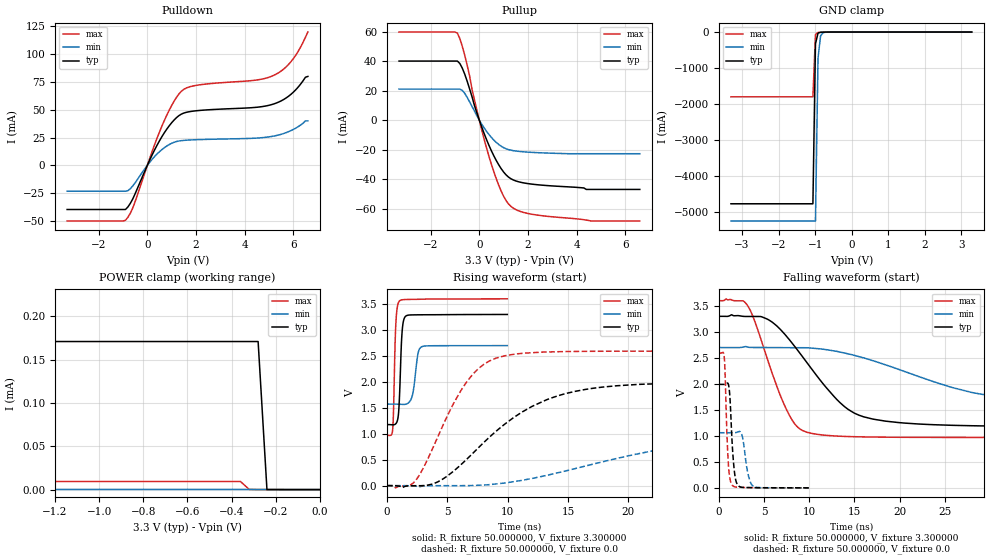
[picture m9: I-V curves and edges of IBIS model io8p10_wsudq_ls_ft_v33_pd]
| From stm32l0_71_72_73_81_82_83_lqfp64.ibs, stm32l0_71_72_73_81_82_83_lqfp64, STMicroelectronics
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|   Model io8p10_wsudq_ls_ft_v33_pd
[Model]  io8p10_wsudq_ls_ft_v33_pd
Model_type I/O
Polarity   Non-Inverting
Enable   Active-Low
Vinl =   0.990000V
Vinh =   2.310000V
Vmeas =  1.650000V
Cref =   50.000000pF
Rref =   100.000000M
Vref =   0.0V
C_comp   2.653200pF   2.620200pF   2.695100pF
[Temperature Range]   25.000000   0.125000k   -40.000000
[Pullup Reference]   3.300000V   2.700000V   3.600000V
[Pulldown Reference]   0.0V   0.0V   0.0V
[POWER Clamp Reference]   3.300000V   2.700000V   3.600000V
[GND Clamp Reference]   0.0V   0.0V   0.0V
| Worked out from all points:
|   slope of the pulldown table from 0 to 0.495 V, typ, clamps not added: 22.6 ohm
|   slope of the pullup table from 0 to 0.495 V, typ, clamps not added: 23.9 ohm
|   GND clamp passes 1 mA (typ) near -0.64 V on its own axis
|   POWER clamp passes 1 mA (typ) near -2.99 V on its own axis
|   rising waveform, R_fixture 50.000000, V_fixture 3.300000: 20-80 % time 213ps typ, 360ps min, 178ps max; typ from 1.18 V to 3.3 V
|   rising waveform, R_fixture 50.000000, V_fixture 0.0: 20-80 % time 6.53ns typ, 13.6ns min, 3.46ns max; typ from 0 V to 1.99 V
|   falling waveform, R_fixture 50.000000, V_fixture 3.300000: 20-80 % time 5.97ns typ, 12.7ns min, 3.28ns max; typ from 3.3 V to 1.18 V
|   falling waveform, R_fixture 50.000000, V_fixture 0.0: 20-80 % time 397ps typ, 565ps min, 319ps max; typ from 1.99 V to 0 V
[Pulldown]
|Voltage   I(typ)   I(min)   I(max)
-3.3V     -39.83mA   -23.37mA   -50.2mA
-900mV    -39.83mA   -23.37mA   -49.53mA
-600mV    -30.28mA   -18.59mA   -38.45mA
100mV     4.867mA    2.821mA    6.48mA
600mV     25.85mA    14.17mA    35.39mA
1V        38.33mA    19.81mA    53.88mA
1.4V      46.1mA     22.18mA    66.72mA
2V        49.07mA    23.02mA    71.93mA
4.4V      52.05mA    24.38mA    76.53mA
5.2V      55.25mA    26.3mA     81.02mA
5.9V      63.83mA    31.17mA    93.18mA
6.6V      80mA       40mA       120mA
[Pullup]
|Voltage   I(typ)   I(min)   I(max)
-3.3V     40.01mA    21.01mA    59.69mA
-900mV    40.01mA    21.01mA    58.93mA
-800mV    38.37mA    21.01mA    55.25mA
-600mV    31.19mA    18.18mA    44.04mA
0V        0A         0A         0A
500mV     -20.88mA   -11.78mA   -30.07mA
900mV     -32.92mA   -17.72mA   -48.15mA
1.3V      -39.75mA   -20.4mA    -58.47mA
1.8V      -42.5mA    -21.48mA   -62.49mA
2.7V      -44.27mA   -22.29mA   -65.04mA
4.6V      -47mA      -22.8mA    -68.41mA
6.6V      -47mA      -22.8mA    -68.41mA
[GND_clamp]
|Voltage   I(typ)   I(min)   I(max)
-3.3V     -4.766A    -5.244A    -1.797A
-1.06V    -4.766A    -5.244A    -1.797A
-990mV    -326.8mA   -5.244A    -68.06mA
-920mV    -29.1mA    -722.2mA   -11.17mA
-850mV    -6.81mA    -104.4mA   -6.691mA
-780mV    -3.567mA   -17.46mA   -4.273mA
-500mV    -68.7uA    -184.5uA   -41.56uA
3.28V     73.95uA    88.62uA    51.48uA
[POWER_clamp]
|Voltage   I(typ)   I(min)   I(max)
-3.28V    3.05A      15.65uA    3.723A
-3.2V     3.05A      1.687uA    3.723A
-2.96V    269.4uA    209.1nA    3.723A
-2.92V    170.9uA    209.1nA    508.5mA
-2.8V     170.9uA    209.1nA    1.296mA
-2.76V    170.9uA    209.1nA    177.1uA
-2.72V    170.9uA    209.1nA    24.25uA
-2.68V    170.9uA    209.1nA    9.362uA
-360mV    170.9uA    209.1nA    9.362uA
-280mV    170.9uA    209.1nA    0A
-240mV    0A         209.1nA    0A
0V        0A         0A         0A
[Ramp]
| variable   typ   min   max
dV/dt_r  1.19406/6.52281n   0.62958/13.57033n   1.55520/3.45923n
dV/dt_f  1.27356/5.95863n   0.65610/12.61269n   1.57835/3.27280n
R_load = 50.000000
[Rising Waveform]
R_fixture= 50.000000
V_fixture= 3.300000
V_fixture_min= 2.700000
V_fixture_max= 3.600000
|time   V(typ)   V(min)   V(max)
0s        1.176V     1.571V     968.9mV
480.5ps   1.172V     1.571V     1.104V
740.7ps   1.196V     1.571V     3.148V
1.021ns   1.641V     1.569V     3.555V
1.241ns   2.93V      1.566V     3.581V
1.542ns   3.264V     1.569V     3.587V
2.102ns   3.29V      1.738V     3.59V
2.543ns   3.292V     2.511V     3.591V
2.883ns   3.293V     2.678V     3.593V
9.97ns    3.299V     2.698V     3.599V
[Rising Waveform]
R_fixture= 50.000000
V_fixture= 0.0
V_fixture_min= 0.0
V_fixture_max= 0.0
|time   V(typ)   V(min)   V(max)
0s        -27.62uV   3.106uV    368.2uV
2.302ns   -1.998mV   -8.931mV   80.74mV
4.204ns   71.67mV    -762.1uV   936.5mV
6.507ns   486.4mV    295.7uV    1.966V
8.008ns   828.7mV    11.96mV    2.335V
9.71ns    1.176V     49.03mV    2.501V
13.61ns   1.689V     218.1mV    2.578V
19.02ns   1.924V     522.6mV    2.591V
31.43ns   1.988V     943.1mV    2.592V
49.85ns   1.99V      1.06V      2.592V
[Falling Waveform]
R_fixture= 50.000000
V_fixture= 3.300000
V_fixture_min= 2.700000
V_fixture_max= 3.600000
|time   V(typ)   V(min)   V(max)
0s        3.299V     2.698V     3.599V
3.103ns   3.296V     2.711V     3.523V
5.305ns   3.249V     2.699V     2.508V
7.407ns   2.93V      2.696V     1.533V
8.509ns   2.693V     2.695V     1.205V
9.71ns    2.416V     2.695V     1.072V
13.91ns   1.56V      2.593V     989.1mV
17.02ns   1.323V     2.447V     977.1mV
30.43ns   1.189V     1.759V     969.2mV
49.85ns   1.176V     1.571V     968.9mV
[Falling Waveform]
R_fixture= 50.000000
V_fixture= 0.0
V_fixture_min= 0.0
V_fixture_max= 0.0
|time   V(typ)   V(min)   V(max)
0s        1.99V      1.06V      2.592V
580.6ps   1.989V     1.06V      2.533V
1.021ns   2.004V     1.06V      530.4mV
1.221ns   1.731V     1.06V      177.2mV
1.441ns   940.2mV    1.06V      59.2mV
1.782ns   225.2mV    1.061V     19.11mV
2.262ns   25.93mV    1.085V     10.49mV
3.283ns   5.049mV    223.2mV    5.21mV
3.824ns   3.748mV    27.3mV     3.888mV
9.97ns    -27.62uV   3.106uV    368.2uV
